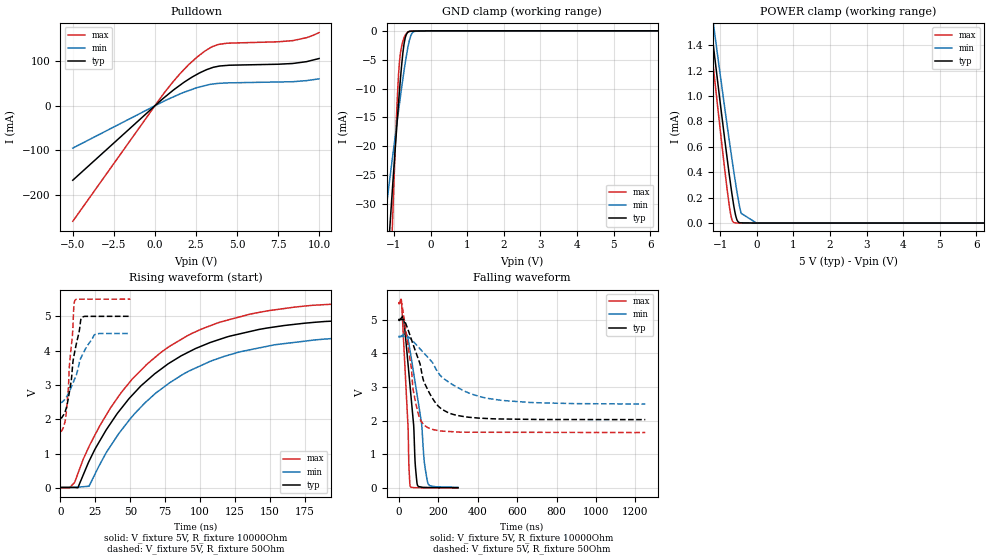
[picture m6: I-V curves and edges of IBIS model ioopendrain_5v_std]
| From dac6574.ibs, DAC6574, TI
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|   ioopendrain_5v_std Model
[Model]   ioopendrain_5v_std
Model_type   I/O_open_drain
Polarity   Non-Inverting
Enable   Active-Low
Vinl = 1.5
Vinh = 3.5
Vmeas = 2.5
Vref = 5.0
Cref = 400pF
Rref = 10000
|   typ   min   max
|   (nom PVT)   (Fast PVT)   (slow PVT)
|Average
C_comp   5.061e-12   5.040e-12   5.094e-12
|ON state : BUFFER OUTPUT TURNED LOW
|C_comp   4.034e-10   3.920e-10   4.419e-10
|OFF state: BUFFER in HIGH IMPEDANCE
|C_comp   5.061e-12   5.040e-12   5.094e-12
| Where nom  PVT is Nominal Process, 5V, 25C
|   Fast PVT is Strong Process,  5.5V, -40C
|   Slow PVT is Weak Process,   4.5V, 105C
[Model spec]
|   typ   min   max
Vinl   1.5   1.35   1.65
Vinh   3.5   3.15   3.85
[Voltage Range]   5   4.5   5.5
|Ambient Temperature   25   105   -40
|Junction Temperature
[Temperature Range]   25   105   -40
[Pullup Reference]   5   4.5   5.5
[Pulldown Reference]   0   0   0
[Power Clamp Reference]   5   4.5   5.5
[GND Clamp Reference]   0   0   0
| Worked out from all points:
|   slope of the pulldown table from 0 to 0.75 V, typ, clamps not added: 31.1 ohm
|   GND clamp passes 1 mA (typ) near -0.68 V on its own axis
|   POWER clamp passes 1 mA (typ) near -1.02 V on its own axis
|   falling waveform, V_fixture 5V, R_fixture 10000Ohm: 20-80 % time 39.1ns typ, 57.1ns min, 25.5ns max; typ from 5 V to 0.015 V
|   rising waveform, V_fixture 5V, R_fixture 10000Ohm: 20-80 % time 70.6ns typ, 71.4ns min, 70.2ns max; typ from 0.015 V to 5 V
|   falling waveform, V_fixture 5V, R_fixture 50Ohm: 20-80 % time 111ns typ, 214ns min, 55.6ns max; typ from 5 V to 2.03 V
|   rising waveform, V_fixture 5V, R_fixture 50Ohm: 20-80 % time 6.86ns typ, 11.3ns min, 4.32ns max; typ from 2.03 V to 5 V
[Pulldown]
|   Voltage   I(typ)   I(min)   I(max)
-5V       -167.6mA   -95.21mA   -260.1mA
632mV     20.56mA    11.88mA    32.24mA
1.567V    47.51mA    27.48mA    73.88mA
2.073V    60.23mA    34.53mA    93.27mA
3.03V     79.48mA    45.34mA    123mA
3.475V    85.81mA    48.85mA    133mA
3.866V    89.13mA    50.56mA    138.4mA
4.41V     91.14mA    51.64mA    141.1mA
7.49V     93.71mA    53.75mA    144.3mA
8.398V    95.44mA    54.36mA    146.9mA
9.239V    99.6mA     56.83mA    153.6mA
10V       106.6mA    60.8mA     165.1mA
[GND Clamp]
|   Voltage   I(typ)   I(min)   I(max)
-5V       -412.1mA   -229.4mA   -786.8mA
-1.266V   -48.89mA   -33.49mA   -75.73mA
-1.101V   -33mA      -25.04mA   -44.62mA
-1.04V    -27.31mA   -21.99mA   -33.44mA
-924.5mV  -16.82mA   -16.27mA   -14.04mA
-886mV    -13.47mA   -14.41mA   -8.932mA
-847.5mV  -10.29mA   -12.56mA   -5.324mA
-725mV    -2.321mA   -6.967mA   -1.233mA
-575mV    -62.02uA   -1.604mA   -142.6uA
-495.5mV  -53.37uA   -326.8uA   -12.8uA
-324.5mV  -34.77uA   -2.562uA   -8.381uA
10V       0A         0A         0A
[POWER Clamp]
|   Voltage   I(typ)   I(min)   I(max)
-5V       10.92mA    10.1mA     11.74mA
-1.335V   1.762mA    1.9mA      1.632mA
-1.265V   1.591mA    1.747mA    1.443mA
-1.238V   1.526mA    1.688mA    1.371mA
-1.15V    1.313mA    1.498mA    1.136mA
-748.5mV  378.2uA    647.3uA    135.5uA
-688mV    251.5uA    526.5uA    38.06uA
-622mV    128.1uA    396.8uA    2.687uA
-535mV    22.14uA    238.1uA    65.67nA
-428mV    1.278uA    76.93uA    28.57nA
-5mV      0A         0A         0A
10V       0A         0A         0A
[Ramp]
R_load = 10000
|   typ   min   max
dV/dt_r   2.99115/7.04898e-08   2.68617/7.10476e-08   3.29376/7.01622e-08
dV/dt_f   2.99115/3.90236e-08   2.68616/5.70956e-08   3.29376/2.54715e-08
[Falling Waveform]
V_fixture = 5V
V_fixture_min = 4.5V
V_fixture_max = 5.5V
R_fixture = 10000Ohm
|   Time   V(typ)   V(min)   V(max)
0s        5V         4.5V       5.5V
13.95ns   5.06V      4.519V     5.449V
25.92ns   4.946V     4.564V     4.114V
46.45ns   3.666V     4.419V     1.788V
50.58ns   3.404V     4.283V     673.9mV
57.03ns   2.993V     4.054V     59.9mV
94.51ns   82.18mV    2.682V     13.49mV
128.8ns   23.91mV    778.3mV    11.55mV
149.1ns   21.84mV    119.6mV    11.39mV
300ns     14.75mV    23.06mV    10.4mV
[Rising Waveform]
V_fixture = 5V
V_fixture_min = 4.5V
V_fixture_max = 5.5V
R_fixture = 10000Ohm
|   Time   V(typ)   V(min)   V(max)
0s        14.75mV    23.05mV    10.4mV
6.439ns   15.87mV    23.72mV    5.059mV
12.47ns   8.346mV    25.59mV    418.5mV
20.46ns   779.7mV    54.77mV    1.209V
33.04ns   1.71V      1.05V      2.144V
51.29ns   2.699V     2.08V      3.168V
77.82ns   3.635V     3.055V     4.118V
114.7ns   4.338V     3.796V     4.835V
195.1ns   4.86V      4.354V     5.354V
500ns     5V         4.5V       5.5V
[Falling Waveform]
V_fixture = 5V
V_fixture_min = 4.5V
V_fixture_max = 5.5V
R_fixture = 50Ohm
|   Time   V(typ)   V(min)   V(max)
0s        5V         4.5V       5.5V
17.42ns   4.998V     4.499V     5.374V
63.83ns   4.401V     4.407V     3.527V
72.07ns   4.261V     4.355V     2.92V
90.41ns   3.957V     4.238V     2.386V
110.6ns   3.583V     4.109V     2.005V
145.3ns   2.931V     3.888V     1.801V
251.1ns   2.236V     3.152V     1.682V
434.4ns   2.07V      2.682V     1.659V
1.25us    2.033V     2.494V     1.65V
[Rising Waveform]
V_fixture = 5V
V_fixture_min = 4.5V
V_fixture_max = 5.5V
R_fixture = 50Ohm
|   Time   V(typ)   V(min)   V(max)
0s        2.033V     2.492V     1.65V
3.947ns   2.297V     2.63V      2.11V
5.663ns   2.616V     2.751V     2.907V
6.435ns   2.807V     2.813V     3.572V
8.599ns   3.52V      3.021V     4.465V
9.654ns   3.846V     3.125V     5.321V
10.35ns   3.995V     3.193V     5.462V
15.5ns    4.976V     3.861V     5.498V
24.28ns   4.998V     4.463V     5.498V
50ns      5V         4.5V       5.5V
